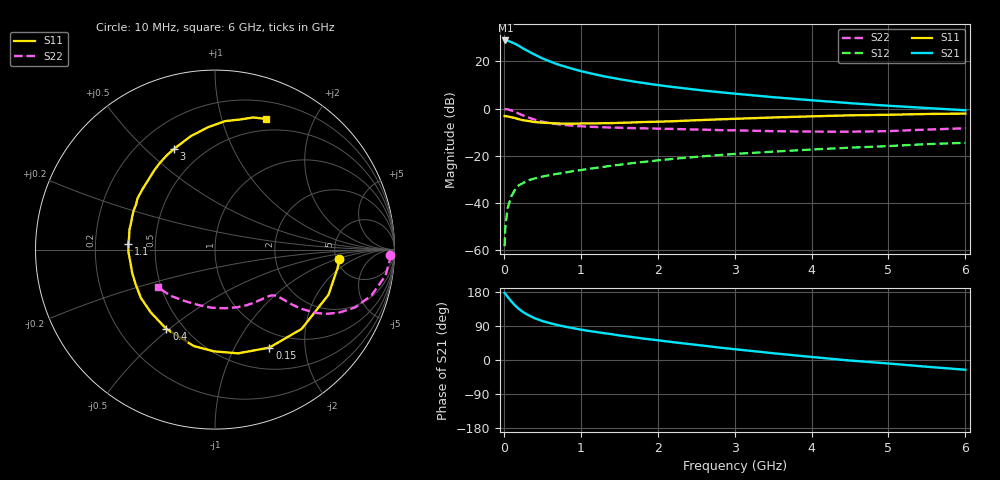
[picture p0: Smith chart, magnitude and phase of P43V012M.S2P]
! SIEMENS Small Signal Semiconductors
! BFP182
! Si NPN RF Bipolar Junction Transistor in SOT143
! VCE = 3 V  IC = 12 mA
! Common Emitter S-Parameters:  March  1996
# GHz  S  MA  R  50
!  f  S11  S21  S12  S22
! GHz  MAG  ANG  MAG  ANG  MAG  ANG  MAG  ANG
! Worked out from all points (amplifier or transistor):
!   36 points, 10 MHz to 6 GHz, reference 50 ohm
!   highest |S21| = 28.9 dB at 20 MHz (marker M1)
!   |S21| within 3 dB of that: start of sweep to 231.3 MHz
!   unconditionally stable (mu >= 1): 1.047 GHz to 5.321 GHz
!   at 250 MHz: K = 0.37, MSG = 28.6 dB, |S12| = -31.6 dB
!   at 1.4 GHz: K = 1.10, MAG = 16.7 dB, |S12| = -24.3 dB
!   at 6 GHz: K = 0.94, MSG = 6.9 dB, |S12| = -14.5 dB
!   S11 on the Smith chart (normalised r, x): 10 MHz: 5.31, -1.09; 150 MHz: 0.78, -1.39; 400 MHz: 0.40, -0.49; 1.1 GHz: 0.35, +0.03; 3 GHz: 0.35, +0.61; 6 GHz: 0.37, +1.40
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0.01  0.6944 -4.4  27.86 177.2  0.0012 88.6  0.9781 -1.6
0.02  0.6906 -8.6  27.88 174.9  0.0031 83.4  0.9759 -3.4
0.05  0.6805 -21.7  27.55 166.4  0.0078 82.7  0.9613 -8.6
0.1  0.6544 -42.5  25.6 154.1  0.014 69.8  0.9085 -16.3
0.15  0.6244 -61.0  23.47 143.1  0.0196 63.3  0.8448 -22.4
0.2  0.592 -77.5  21.21 133.9  0.0238 57.8  0.7758 -26.9
0.25  0.5667 -90.7  18.9 126.5  0.0262 53.9  0.7142 -30.1
0.3  0.5501 -102.4  17.04 120.5  0.0294 51.6  0.6615 -32.2
0.4  0.5184 -121.5  13.96 110.3  0.0328 48.1  0.5819 -34.5
0.5  0.5005 -135.6  11.62 102.9  0.036 45.7  0.5269 -35.5
0.6  0.493 -146.8  10.01 97.2  0.0388 45.7  0.4904 -35.9
0.7  0.4824 -156.6  8.657 92.2  0.0413 45.8  0.4653 -36.2
0.9  0.4767 -171.2  6.924 84.1  0.0471 46.8  0.4316 -36.8
1.1  0.4839 176.5  5.716 76.8  0.0524 47.2  0.4126 -38.3
1.5  0.4964 158.5  4.217 64.9  0.064 47.5  0.3923 -42.2
1.8  0.5174 146.6  3.519 56.9  0.0732 47.3  0.3811 -46.3
2.2  0.5375 133.7  2.865 47.0  0.0854 45.2  0.3696 -52.8
3  0.6054 112.3  2.073 28.5  0.1089 39.9  0.3446 -68.9
3.5  0.6469 101.9  1.743 17.9  0.1217 35.9  0.3312 -80.8
4.5  0.7183 85.4  1.302 -1.4  0.1479 28.3  0.3225 -107.5
5.5  0.7667 73.8  1.026 -17.8  0.176 20.6  0.3578 -134.2
6  0.782 68.5  0.92 -25.7  0.1874 15.8  0.3813 -146.8
